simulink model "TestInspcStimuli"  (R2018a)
settings: Solver=VariableStepAuto  StartTime=0.0  StopTime=4  RelTol=1e-3
PreLoadFcn:
  | inspcStimuli.TestInspcStimuli_init();
StartFcn:
  | inspcStimuli.TestInspcStimuli_init();
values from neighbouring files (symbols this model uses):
  Tstep = 0.0001    [TestInspcStimuli_init.m]
libraries: lib_Inspc x3

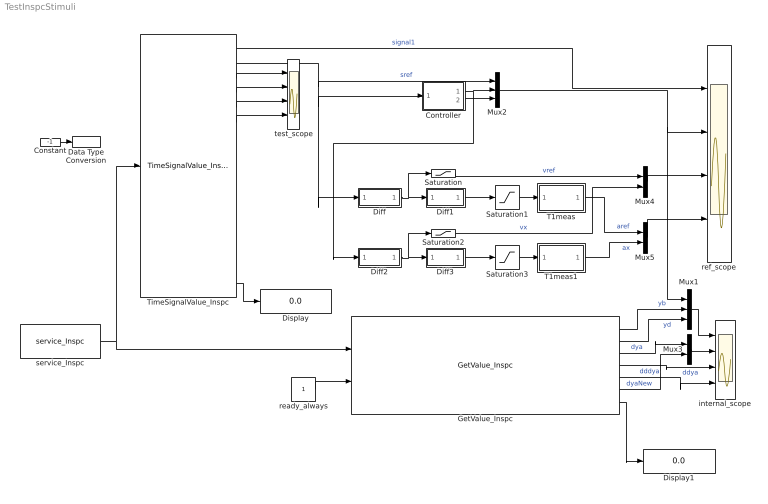
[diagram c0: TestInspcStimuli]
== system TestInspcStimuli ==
  Constant : Constant  Value=-1  OutDataTypeStr=int32
  Controller : Subsystem  mask{TI=0.01}
      mask prompts: TI "Tintg"
  Data Type Conversion : DataTypeConversion  OutDataTypeStr=uint32
  Diff : Subsystem
  Diff1 : Subsystem
  Diff2 : Subsystem
  Diff3 : Subsystem
  Display : Display
  Display1 : Display
  GetValue_Inspc : lib_Inspc/GetValue_Inspc  Tstep=Tstep  path1='timeSignals.thiz$TimeSignals_Inspc.curr[1].yb[0]'  path2='timeSignals.thiz$TimeSignals_Inspc.curr[1].yd[0]'  path3='timeSignals.thiz$TimeSignals_Inspc.curr[1].dya[0]'  path4='timeSignals.thiz$TimeSignals_Inspc.curr[1].ddya[0]'  path5='timeSignals.thiz$TimeSignals_Inspc.curr[1].dddya[0]'  path6='timeSignals.thiz$TimeSignals_Inspc.curr[1].dyaNew[0]'
  Mux1 : Mux  Inputs=3
  Mux2 : Mux  Inputs=3
  Mux3 : Mux  Inputs=2
  Mux4 : Mux  Inputs=2
  Mux5 : Mux  Inputs=2
  Saturation : Saturate  UpperLimit=50  LowerLimit=-50
  Saturation1 : Saturate  UpperLimit=500  LowerLimit=-500
  Saturation2 : Saturate  UpperLimit=50  LowerLimit=-50
  Saturation3 : Saturate  UpperLimit=500  LowerLimit=-500
  T1meas : Subsystem  mask{T1=0.001}
  T1meas1 : Subsystem  mask{T1=0.001}
  TimeSignalValue_Inspc : lib_Inspc/TimeSignalValue_Inspc  Description=|  Tstep=Tstep  filepath=timeSignalFilepath  nameRefl='timeSignals'  nrofStimuli=25  n1='signal1'  n2='sref'  n3='6:vector'  n4='C:complex'  n5='C3:complexvector'  n6=''  n7=''  n8=''  n9=''  n10=''  n11=''  n12=''  n13=''  n14='dyatarget'  n15='dya'  n16='ft1'
      | A combined stimuli and inspector function block.
      | Stimuli file path: file contains stimuli in form:
      |   %time:0: stimuli.namex = 5000.0, stimuli.namey = 50.0 -10; 
      | Name in reflection-tree: Name of this function block for stimuli and inspector access
      | name1..12: output type and name, base type is single always.
      | C2:namexy  A complex array of 2 elements
      | 6:namexy An array of 6 elements (max).
      | C:namexy  A 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
  internal_scope : Scope  NumInputPorts=4
  ready_always : Constant  OutDataTypeStr=int32
  ref_scope : Scope  NumInputPorts=4
  service_Inspc : lib_Inspc/service_Inspc  Tstep=Tstep  IpPort='UDP:0.0.0.0:60094'
  test_scope : Scope  NumInputPorts=4
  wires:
  Constant/1 -> Data Type Conversion/1
  TimeSignalValue_Inspc/17 -> Display/1
  TimeSignalValue_Inspc/2 -> Mux2/1, Controller/1(In1), Diff/1(In1)  "sref"
  GetValue_Inspc/1 -> Mux1/2  "yb"
  ready_always/1 -> GetValue_Inspc/2
  GetValue_Inspc/7 -> Display1/1
  GetValue_Inspc/2 -> Mux1/3  "yd"
  GetValue_Inspc/3 -> Mux3/1  "dya"
  Mux1/1 -> internal_scope/1
  GetValue_Inspc/5 -> internal_scope/4  "dddya"
  Controller/1(Out1) -> Diff2/1(In1), Mux2/2
  Mux2/1 -> Mux1/1, ref_scope/2
  GetValue_Inspc/4 -> internal_scope/3  "ddya"
  Mux3/1 -> internal_scope/2
  GetValue_Inspc/6 -> Mux3/2  "dyaNew"
  Diff/1(Out1) -> Diff1/1(In1), Saturation/1
  Diff1/1(Out1) -> Saturation1/1
  TimeSignalValue_Inspc/1 -> ref_scope/1  "signal1"
  T1meas/1(Out2) -> Mux5/1  "aref"
  Saturation/1 -> Mux4/1  "vref"
  Saturation1/1 -> T1meas/1(In2)
  Controller/2(Out2) -> Mux2/3
  Mux4/1 -> ref_scope/3
  Mux5/1 -> ref_scope/4
  Diff2/1(Out1) -> Diff3/1(In1), Saturation2/1
  Saturation3/1 -> T1meas1/1(In2)
  Diff3/1(Out1) -> Saturation3/1
  Saturation2/1 -> Mux4/2  "vx"
  T1meas1/1(Out2) -> Mux5/2  "ax"
  TimeSignalValue_Inspc/3 -> test_scope/1
  TimeSignalValue_Inspc/4 -> test_scope/2
  TimeSignalValue_Inspc/5 -> test_scope/3
  TimeSignalValue_Inspc/6 -> test_scope/4
  service_Inspc/1 -> TimeSignalValue_Inspc/1, GetValue_Inspc/1

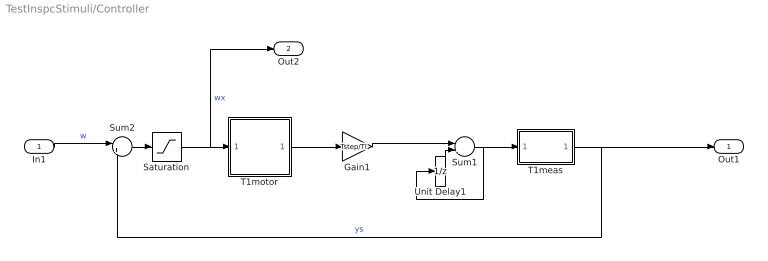
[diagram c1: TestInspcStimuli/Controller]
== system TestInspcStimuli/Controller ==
  In1 : Inport
  Gain1 : Gain  Gain=Tstep/TI
  Saturation : Saturate
  Sum1 : Sum  Inputs=|++
  Sum2 : Sum  Inputs=|+-
  T1meas : Subsystem  mask{T1=0.01}
  T1motor : Subsystem  mask{T1=0.05}
  Unit Delay1 : UnitDelay  SampleTime=-1
  Out1 : Outport
  Out2 : Outport  Port=2
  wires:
  T1meas/1(Out2) -> Sum2/2, Out1/1  "ys"
  In1/1 -> Sum2/1  "w"
  Unit Delay1/1 -> Sum1/2
  Sum1/1 -> T1meas/1(In2), Unit Delay1/1
  Sum2/1 -> Saturation/1
  Gain1/1 -> Sum1/1
  T1motor/1(Out2) -> Gain1/1
  Saturation/1 -> Out2/1, T1motor/1(In2)  "wx"

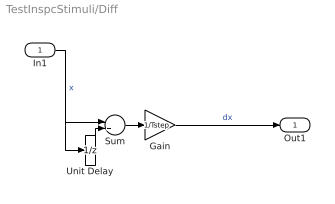
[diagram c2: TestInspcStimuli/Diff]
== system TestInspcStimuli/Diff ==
  In1 : Inport
  Gain : Gain  Gain=1/Tstep
  Sum : Sum  Inputs=|+-
  Unit Delay : UnitDelay  SampleTime=-1
  Out1 : Outport
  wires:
  Gain/1 -> Out1/1  "dx"
  In1/1 -> Unit Delay/1, Sum/1  "x"
  Unit Delay/1 -> Sum/2
  Sum/1 -> Gain/1

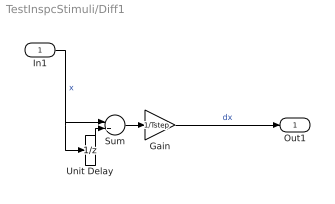
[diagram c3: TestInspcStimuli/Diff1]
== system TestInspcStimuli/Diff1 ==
  In1 : Inport
  Gain : Gain  Gain=1/Tstep
  Sum : Sum  Inputs=|+-
  Unit Delay : UnitDelay  SampleTime=-1
  Out1 : Outport
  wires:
  Gain/1 -> Out1/1  "dx"
  In1/1 -> Unit Delay/1, Sum/1  "x"
  Unit Delay/1 -> Sum/2
  Sum/1 -> Gain/1

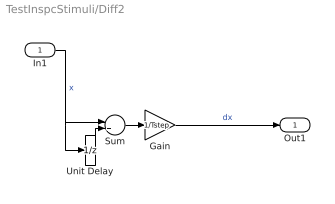
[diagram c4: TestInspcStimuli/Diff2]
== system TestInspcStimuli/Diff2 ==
  In1 : Inport
  Gain : Gain  Gain=1/Tstep
  Sum : Sum  Inputs=|+-
  Unit Delay : UnitDelay  SampleTime=-1
  Out1 : Outport
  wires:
  Gain/1 -> Out1/1  "dx"
  In1/1 -> Unit Delay/1, Sum/1  "x"
  Unit Delay/1 -> Sum/2
  Sum/1 -> Gain/1

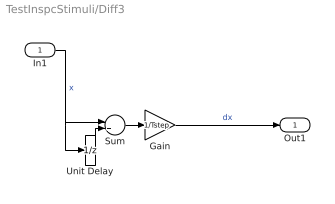
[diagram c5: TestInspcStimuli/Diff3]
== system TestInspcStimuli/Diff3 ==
  In1 : Inport
  Gain : Gain  Gain=1/Tstep
  Sum : Sum  Inputs=|+-
  Unit Delay : UnitDelay  SampleTime=-1
  Out1 : Outport
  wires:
  Gain/1 -> Out1/1  "dx"
  In1/1 -> Unit Delay/1, Sum/1  "x"
  Unit Delay/1 -> Sum/2
  Sum/1 -> Gain/1

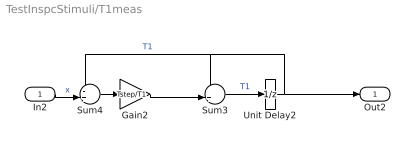
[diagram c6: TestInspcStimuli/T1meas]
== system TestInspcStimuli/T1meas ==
  In2 : Inport
  Gain2 : Gain  Gain=Tstep/T1
  Sum3 : Sum  Inputs=++|
  Sum4 : Sum  Inputs=-+|
  Unit Delay2 : UnitDelay  SampleTime=-1
  Out2 : Outport
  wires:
  Sum4/1 -> Gain2/1
  In2/1 -> Sum4/2  "x"
  Sum3/1 -> Unit Delay2/1  "T1"
  Gain2/1 -> Sum3/2
  Unit Delay2/1 -> Sum4/1, Sum3/1, Out2/1  "T1"

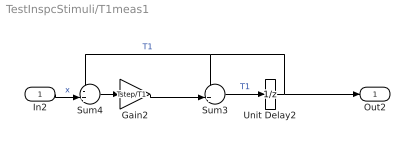
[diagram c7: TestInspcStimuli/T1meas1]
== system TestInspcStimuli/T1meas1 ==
  In2 : Inport
  Gain2 : Gain  Gain=Tstep/T1
  Sum3 : Sum  Inputs=++|
  Sum4 : Sum  Inputs=-+|
  Unit Delay2 : UnitDelay  SampleTime=-1
  Out2 : Outport
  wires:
  Sum4/1 -> Gain2/1
  In2/1 -> Sum4/2  "x"
  Sum3/1 -> Unit Delay2/1  "T1"
  Gain2/1 -> Sum3/2
  Unit Delay2/1 -> Sum4/1, Sum3/1, Out2/1  "T1"

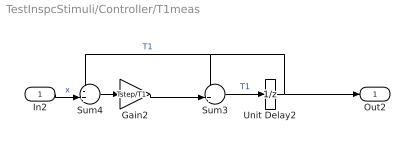
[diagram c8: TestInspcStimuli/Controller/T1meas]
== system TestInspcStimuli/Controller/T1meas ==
  In2 : Inport
  Gain2 : Gain  Gain=Tstep/T1
  Sum3 : Sum  Inputs=++|
  Sum4 : Sum  Inputs=-+|
  Unit Delay2 : UnitDelay  SampleTime=-1
  Out2 : Outport
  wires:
  Sum4/1 -> Gain2/1
  In2/1 -> Sum4/2  "x"
  Sum3/1 -> Unit Delay2/1  "T1"
  Gain2/1 -> Sum3/2
  Unit Delay2/1 -> Sum4/1, Sum3/1, Out2/1  "T1"

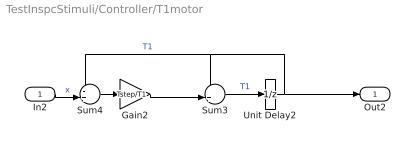
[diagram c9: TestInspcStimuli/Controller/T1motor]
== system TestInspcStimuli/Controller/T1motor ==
  In2 : Inport
  Gain2 : Gain  Gain=Tstep/T1
  Sum3 : Sum  Inputs=++|
  Sum4 : Sum  Inputs=-+|
  Unit Delay2 : UnitDelay  SampleTime=-1
  Out2 : Outport
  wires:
  Sum4/1 -> Gain2/1
  In2/1 -> Sum4/2  "x"
  Sum3/1 -> Unit Delay2/1  "T1"
  Gain2/1 -> Sum3/2
  Unit Delay2/1 -> Sum4/1, Sum3/1, Out2/1  "T1"
